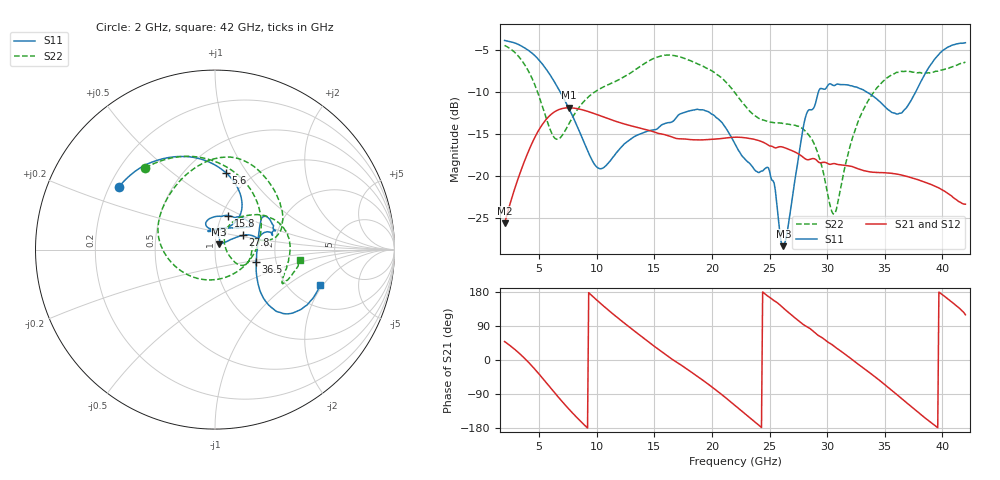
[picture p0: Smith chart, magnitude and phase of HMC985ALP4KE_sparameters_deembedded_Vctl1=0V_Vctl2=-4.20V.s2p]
!s2p File: Measurements: S11, S21, S12, S22
# GHz S dB R 50.0
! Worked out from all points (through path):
!   401 points, 2 GHz to 42 GHz, reference 50 ohm
!   highest |S21| = -11.89 dB at 7.6 GHz (marker M1); lowest = -25.7 dB at 2 GHz (marker M2)
!   lowest |S11| = -28.4 dB at 26.2 GHz (marker M3), VSWR 1.08, Z = 52.3 + j3.17 ohm
!   |S11| at or under -10 dB: 6.822 GHz to 29.25 GHz (22.43 GHz wide, 124 % of centre); 33.42 GHz to 37.69 GHz (4.27 GHz wide, 12 % of centre)
!   |S22| runs from -24.5 to -4.5 dB; largest |S21 - S12| = 0.00021
!   S11 on the Smith chart (normalised r, x): 2 GHz: 0.24, +0.28; 5.6 GHz: 0.76, +0.80; 15.8 GHz: 1.07, +0.42; 27.8 GHz: 1.34, +0.22; 36.5 GHz: 1.57, -0.23; 42 GHz: 2.95, -1.89
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2  -3.88 147.0  -25.66 48.6  -25.67 48.6  -4.47 130.5
3.6  -4.66 120.3  -18.70 8.3  -18.70 8.3  -6.48 84.9
4.7  -5.80 99.5  -15.21 -26.9  -15.22 -26.9  -9.43 43.4
5.6  -7.28 81.9  -13.29 -59.1  -13.30 -59.1  -13.08 -3.8
6.5  -9.22 66.5  -12.25 -92.1  -12.25 -92.1  -15.63 -69.2
7.6  -12.03 54.8  -11.89 -130.2  -11.90 -130.2  -13.76 -136.0
8.7  -15.38 55.0  -12.12 -164.8  -12.12 -164.8  -11.43 -170.4
10.4  -19.14 89.6  -12.89 147.4  -12.90 147.4  -9.54 162.3
15.4  -14.22 75.7  -14.96 27.3  -14.97 27.3  -5.79 86.8
15.8  -13.83 68.7  -15.06 18.4  -15.07 18.4  -5.66 81.7
19.4  -12.23 33.3  -15.71 -57.6  -15.71 -57.6  -7.08 34.7
22  -16.19 51.2  -15.40 -119.9  -15.41 -119.9  -10.12 9.9
24.9  -19.04 104.7  -16.36 167.4  -16.36 167.4  -13.54 13.2
26.2  -28.37 52.5  -16.60 137.0  -16.60 137.0  -13.77 -2.9
27.8  -15.23 27.2  -17.66 96.5  -17.66 96.5  -14.32 -25.0
28.7  -12.11 12.6  -17.95 78.4  -17.95 78.3  -15.71 -31.8
30.6  -9.26 19.5  -18.54 36.5  -18.54 36.4  -24.54 18.0
32.8  -9.59 33.9  -19.21 -13.5  -19.21 -13.5  -13.13 52.9
35.4  -12.22 11.7  -19.68 -74.8  -19.68 -74.8  -8.16 20.9
36.5  -12.47 -16.7  -19.91 -102.7  -19.91 -102.7  -7.56 6.9
39.5  -5.85 -43.7  -21.31 -176.3  -21.32 -176.4  -7.54 -26.3
42  -4.15 -18.6  -23.37 119.4  -23.39 119.3  -6.43 -6.9
